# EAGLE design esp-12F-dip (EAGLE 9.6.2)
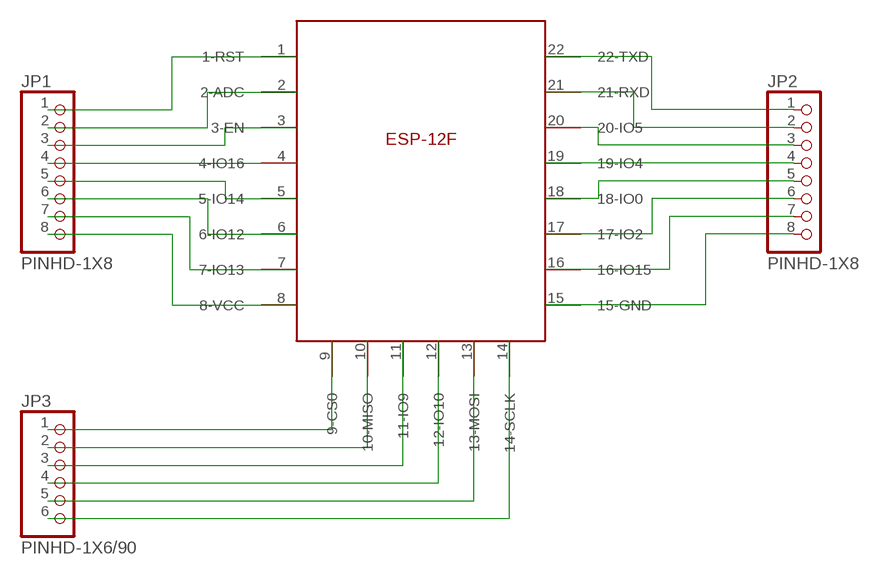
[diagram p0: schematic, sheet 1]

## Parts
JP1  PINHD-1X8  [1X08]
JP2  PINHD-1X8  [1X08]
JP3  PINHD-1X6/90  [1X06/90]
U$1  ESP-12F  [ESP-12F]

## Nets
N$1: JP1.5 U$1.5(5-IO14)
N$2: JP1.3 U$1.3(3-EN)
N$3: JP1.2 U$1.2(2-ADC)
N$4: JP1.4 U$1.4(4-IO16)
N$5: JP1.1 U$1.1(1-RST)
N$6: JP1.6 U$1.6(6-IO12)
N$7: JP1.7 U$1.7(7-IO13)
N$8: JP1.8 U$1.8(8-VCC)
N$9: JP3.1 U$1.9(9-CS0)
N$10: JP3.2 U$1.10(10-MISO)
N$11: JP3.3 U$1.11(11-IO9)
N$12: JP3.4 U$1.12(12-IO10)
N$13: JP3.5 U$1.13(13-MOSI)
N$14: JP3.6 U$1.14(14-SCLK)
N$15: JP2.4 U$1.19(19-IO4)
N$16: JP2.5 U$1.18(18-IO0)
N$17: JP2.6 U$1.17(17-IO2)
N$18: JP2.3 U$1.20(20-IO5)
N$19: JP2.2 U$1.21(21-RXD)
N$20: JP2.1 U$1.22(22-TXD)
N$21: JP2.7 U$1.16(16-IO15)
N$22: JP2.8 U$1.15(15-GND)

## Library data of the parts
JP1 JP2 = Connector:PINHD-1X8: PIN HEADER; CATEGORY: CONNECTOR; SUB-CATEGORY: PIN-HEADER
JP3 = Connector:PINHD-1X6: PIN HEADER; CATEGORY: CONNECTOR; SUB-CATEGORY: PIN-HEADER
U$1 = _My_:ESP-12F

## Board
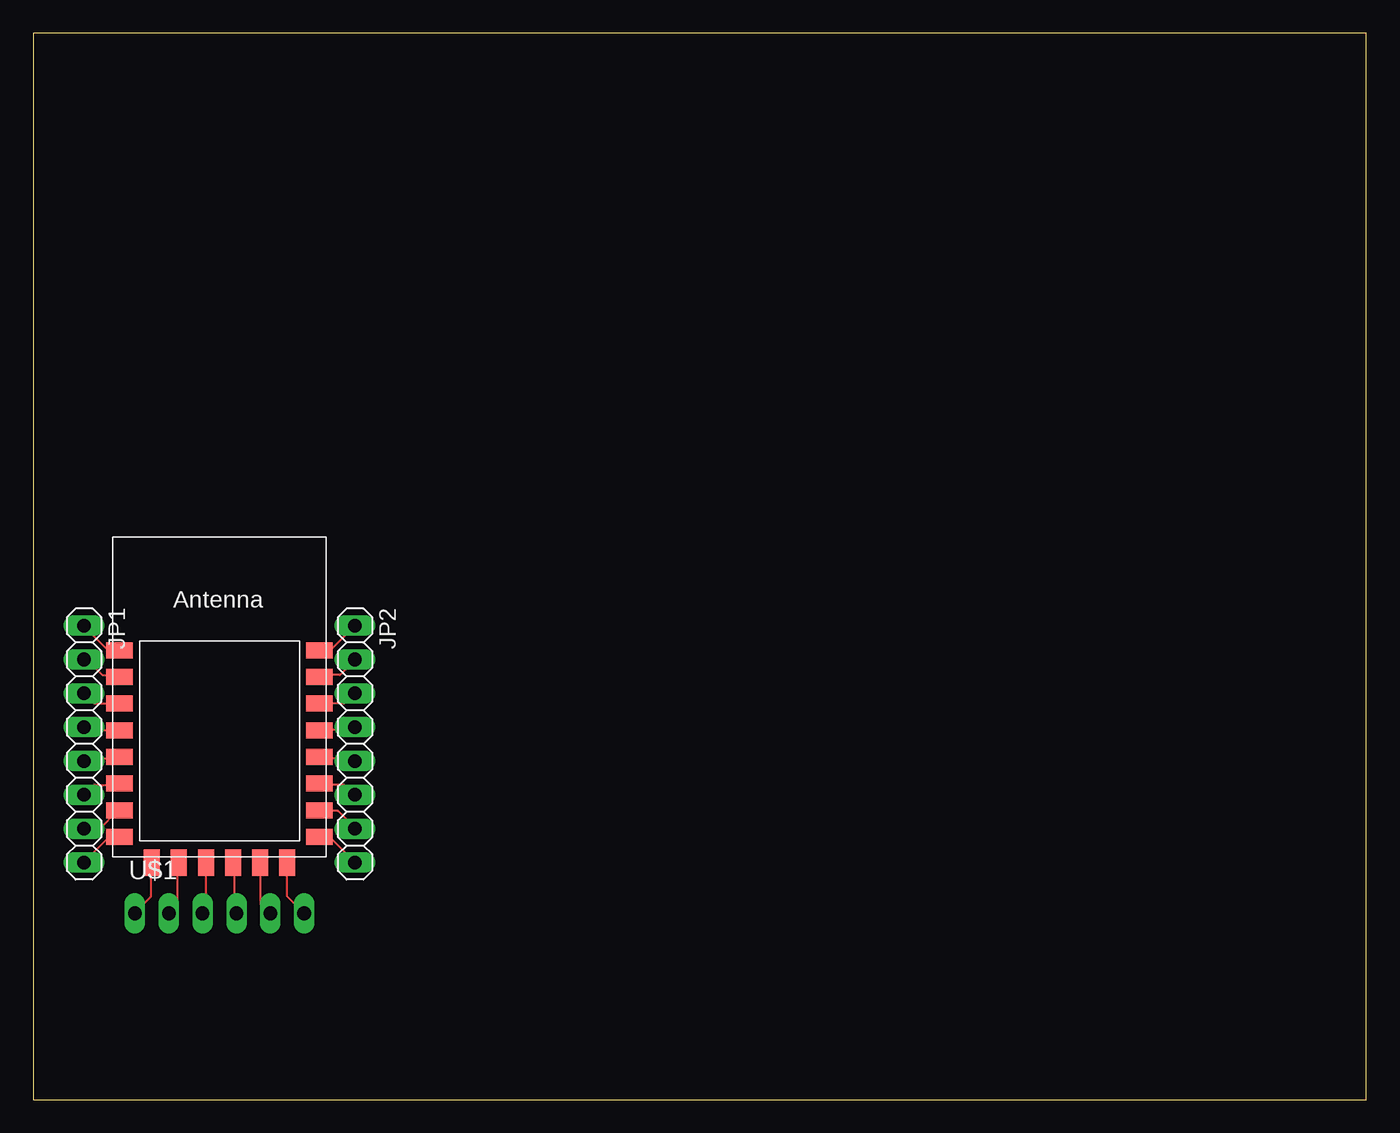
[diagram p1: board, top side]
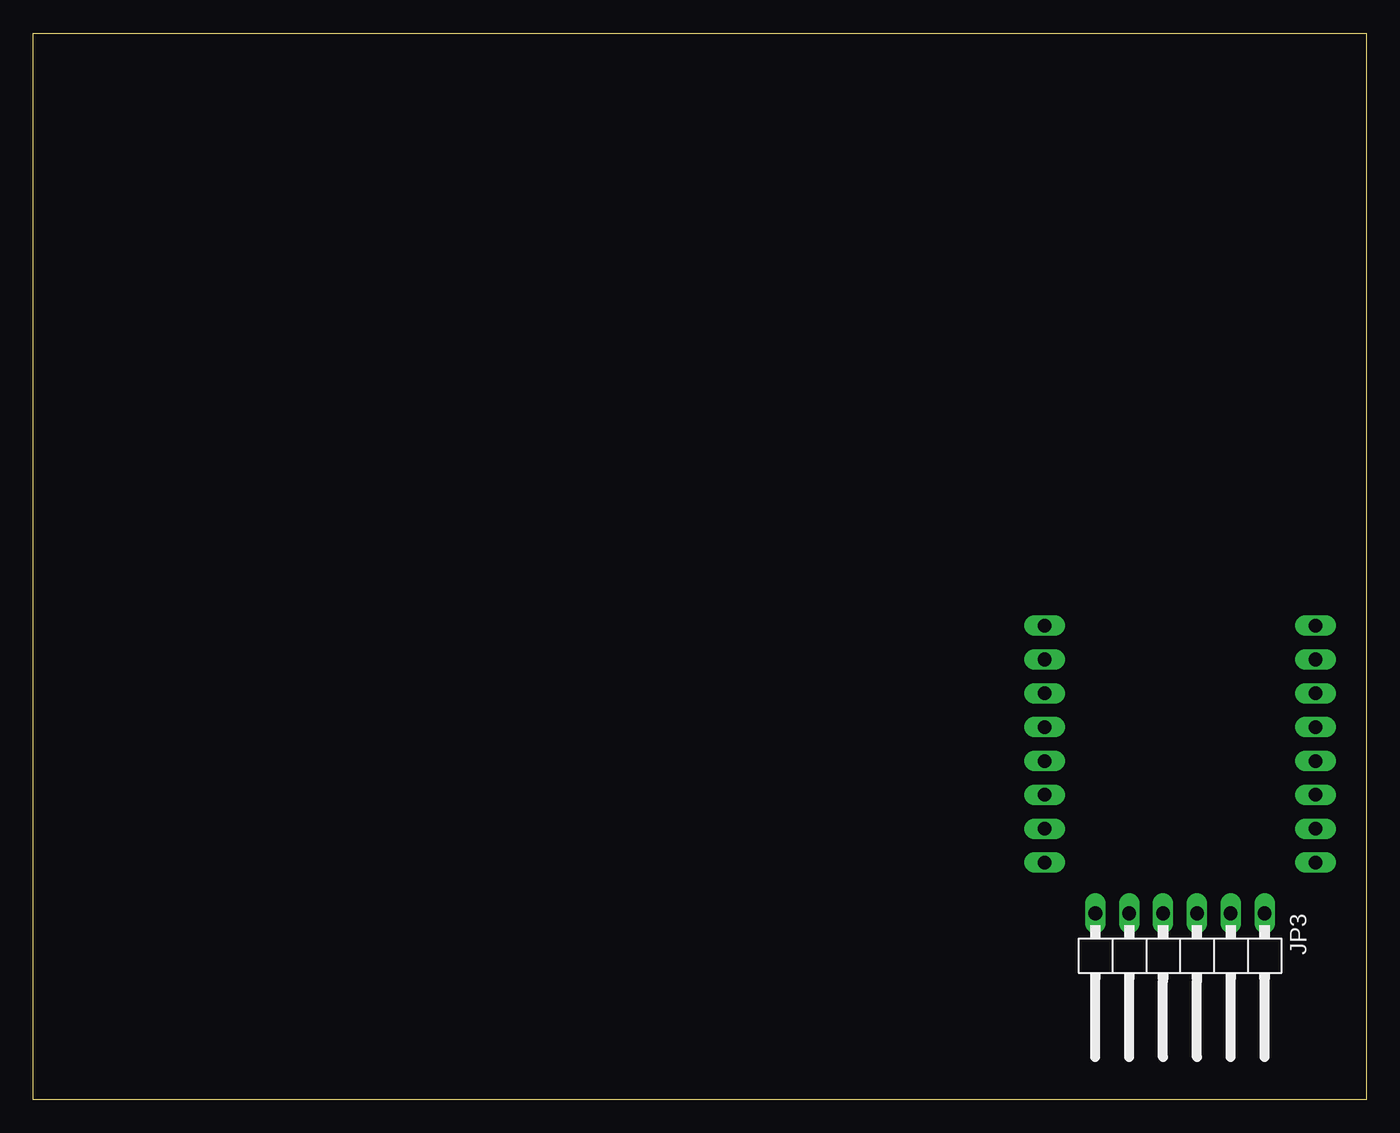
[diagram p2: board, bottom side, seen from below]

Size 100 x 80 mm. Coordinates in mm from the lower left corner, seen from the top.
Outline: 0,0 100,0 100,80 0,80 0,0
Copper layers (1*16): Top 0.035mm / dielectric 1.5mm / Bottom 0.035mm
Design rules "default": minimum track width 6mil, minimum drill 0.35mm, track to track 6mil, track to pad 6mil, pad to pad 6mil, via to via 6mil, smd to smd 6mil, copper to edge 40mil, drill to drill 6mil, minimum pad ring 10mil, minimum via ring 8mil, stop-mask expansion 4mil, vias tented up to drill 0mil, thermal gap 10mil

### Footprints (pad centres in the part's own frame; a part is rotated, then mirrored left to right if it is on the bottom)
1X08 = drill 1.016 long: 1 -8.89,0; 2 -6.35,0; 3 -3.81,0; 4 -1.27,0; 5 1.27,0; 6 3.81,0; 7 6.35,0; 8 8.89,0
1X06/90 = drill 1.016 long: 1 -6.35,-3.81; 2 -3.81,-3.81; 3 -1.27,-3.81; 4 1.27,-3.81; 5 3.81,-3.81; 6 6.35,-3.81
ESP-12F = smd 2 x 1.2: 1 -7.5,4.5; 2 -7.5,2.5; 3 -7.5,0.5; 4 -7.5,-1.5; 5 -7.5,-3.5; 6 -7.5,-5.5; 7 -7.5,-7.5; 8 -7.5,-9.5; 15 7.5,-9.5; 16 7.5,-7.5; 17 7.5,-5.5; 18 7.5,-3.5; 19 7.5,-1.5; 20 7.5,0.5; 21 7.5,2.5; 22 7.5,4.5 | smd 1.2 x 2: 9 -5.08,-11.43; 10 -3.048,-11.43; 11 -1.016,-11.43; 12 1.016,-11.43; 13 3.048,-11.43; 14 5.08,-11.43

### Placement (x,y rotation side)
JP1  3.81,26.67 270 top
JP2  24.13,26.67 270 top
JP3  13.97,10.16 180 bottom
U$1  13.97,29.21 0 top

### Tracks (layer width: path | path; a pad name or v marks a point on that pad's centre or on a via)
N$1
  Top 0.152: 3.96,25.6 3.81,25.45 JP1.5 3.96,25.6 | 3.96,25.6 6.4,25.6 U$1.5
N$2
  Top 0.152: JP1.3 4.57,29.72 6.4,29.72 U$1.3
N$3
  Top 0.152: 3.91,33.12 JP1.2 3.96,33.07 5.18,31.85 6.4,31.85 U$1.2
N$4
  Top 0.152: 3.96,27.74 3.81,27.89 JP1.4 3.96,27.74 | 3.96,27.74 6.4,27.74 U$1.4
N$5
  Top 0.152: U$1.1 6.4,33.83 5.49,33.83 3.81,35.51 JP1.1
N$6
  Top 0.152: JP1.6 4.57,23.62 6.4,23.62 U$1.6
N$7
  Top 0.152: 3.81,20.37 JP1.7 4.98,20.32 6.3,21.64 6.4,21.64 U$1.7
N$8
  Top 0.152: U$1.8 6.4,19.66 5.64,19.66 3.81,17.83 JP1.8
N$9
  Top 0.152: U$1.9 8.84,17.68 8.84,15.24 7.62,14.02 JP3.1
N$10
  Top 0.152: JP3.2 10.82,14.63 10.82,17.68 U$1.10
N$11
  Top 0.152: U$1.11 12.95,14.17 12.8,14.02 JP3.3
N$12
  Top 0.152: U$1.12 15.09,17.68 15.09,14.17 15.24,14.02 JP3.4
N$13
  Top 0.152: U$1.13 17.07,17.68 17.07,14.63 17.68,14.02 JP3.5
N$14
  Top 0.152: U$1.14 19.05,15.24 JP3.6
N$15
  Top 0.152: JP2.4 23.93,27.74 21.49,27.74 U$1.19
N$16
  Top 0.152: JP2.5 23.93,25.6 21.49,25.6 U$1.18
N$17
  Top 0.152: U$1.17 21.49,23.62 23.32,23.62 24.08,22.86 JP2.6
N$18
  Top 0.152: U$1.20 21.49,29.72 23.32,29.72 24.08,30.48 JP2.3
N$19
  Top 0.152: U$1.21 21.49,31.85 23.01,31.85 24.08,32.92 JP2.2
N$20
  Top 0.152: JP2.1 22.4,33.83 21.49,33.83 U$1.22
N$21
  Top 0.152: 21.59,21.64 21.49,21.64 U$1.16 21.64,21.64 22.86,21.64 24.08,20.42 JP2.7
N$22
  Top 0.152: JP2.8 22.25,19.66 21.49,19.66 U$1.15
